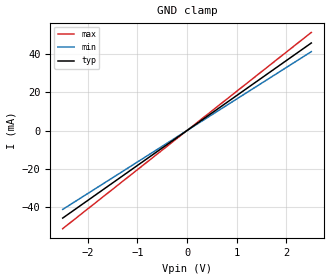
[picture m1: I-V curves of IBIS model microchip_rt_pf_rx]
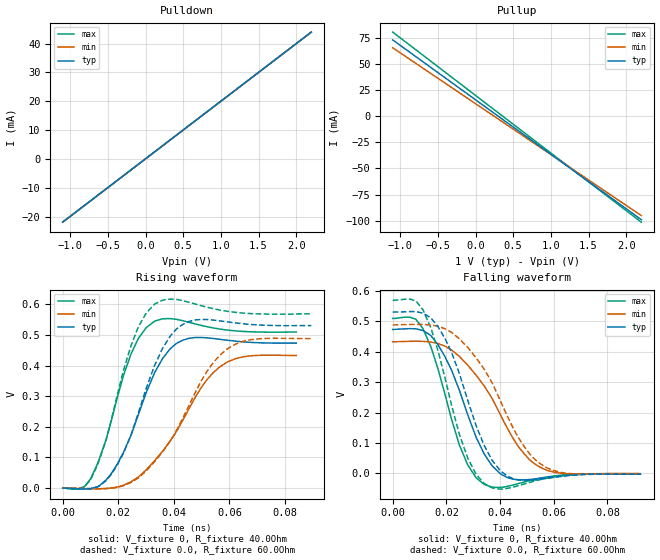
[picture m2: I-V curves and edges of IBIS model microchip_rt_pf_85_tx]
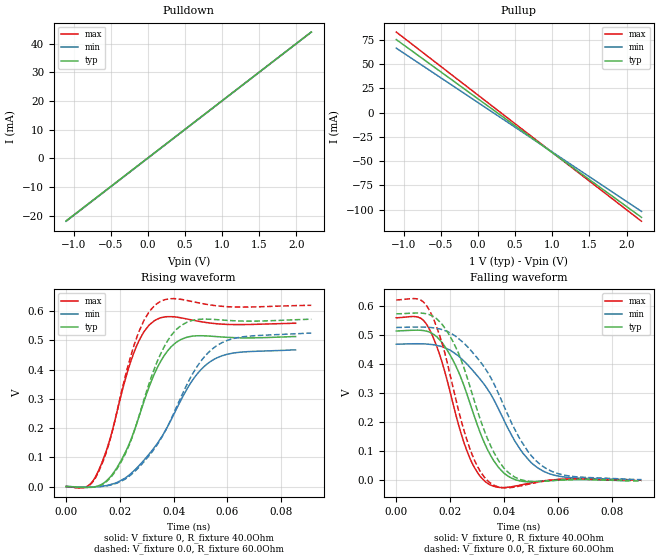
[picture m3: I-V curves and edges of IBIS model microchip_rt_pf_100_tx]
|   Microchip RT PF SerDes IBIS-AMI Model
[IBIS Ver]   6.0
[Disclaimer] THIS IBIS MODEL HAS BEEN CREATED BY THE SIGNAL
   INTEGRITY SOFTWARE SPICE WRAPPING PROCESS.
   THESE IBIS MODELS AREPROVIDED "AS IS" WITH NO
   WARRANTY WHATSOEVER AND SIGNAL INTEGRITY SOFTWARE
   SPECIFICALLY DISCLAIMS ANY IMPLIED WARRANTIES OF
   MERCHANTABILITY, FITNESS FOR A PARTICULAR PURPOSE,
   OR AGAINST INFRINGEMENT.
[File Name]  microchip_rt_pf.ibs
[Date]   Sep/20/2022
[File Rev]   1.0
[Source]   SPISim LLC, Generated by SPIBPro
[Notes]   Revision 1.0 - Sep/20/2022
|   - Passes IBISCHK6 V6.1.4 with 0 Errors and 0 Warnings.
[Copyright]  Copyright 2022, SPISim LLC, All Rights Reserved.
|   COMPONENT: microchip_rt_pf_serdes
[Component] microchip_rt_pf_serdes
[Manufacturer]  microchip
[Package]
R_pkg   0.001m  NA NA
L_pkg   0.000nH NA NA
C_pkg   0.000pF NA NA
[Pin] signal_name   model_name   R_pin L_pin C_pin
1   microchip_rt_pf_rx_p   microchip_rt_pf_rx   NA   NA   NA
2   microchip_rt_pf_rx_n   microchip_rt_pf_rx   NA   NA   NA
3   microchip_rt_pf_85_tx_p   microchip_rt_pf_85_tx   NA   NA   NA
4   microchip_rt_pf_85_tx_n   microchip_rt_pf_85_tx   NA   NA   NA
5   microchip_rt_pf_100_tx_p   microchip_rt_pf_100_tx   NA   NA   NA
6   microchip_rt_pf_100_tx_n   microchip_rt_pf_100_tx   NA   NA   NA
7   microchip_rt_pf_150_tx_p   microchip_rt_pf_150_tx   NA   NA   NA
8   microchip_rt_pf_150_tx_n   microchip_rt_pf_150_tx   NA   NA   NA
9   microchip_rt_pf_180_tx_p   microchip_rt_pf_180_tx   NA   NA   NA
10   microchip_rt_pf_180_tx_n   microchip_rt_pf_180_tx   NA   NA   NA
11   microchip_rt_pf_150_400tx_p   microchip_rt_pf_150_400_tx  NA   NA   NA
12   microchip_rt_pf_150_400tx_n   microchip_rt_pf_150_400_tx  NA   NA   NA
13   microchip_rt_pf_150_800tx_p   microchip_rt_pf_150_800_tx  NA   NA   NA
14   microchip_rt_pf_150_800tx_n   microchip_rt_pf_150_800_tx  NA   NA   NA
15   microchip_rt_pf_180_400tx_p   microchip_rt_pf_180_400_tx  NA   NA   NA
16   microchip_rt_pf_180_400tx_n   microchip_rt_pf_180_400_tx  NA   NA   NA
17   microchip_rt_pf_180_800tx_p   microchip_rt_pf_180_800_tx  NA   NA   NA
18   microchip_rt_pf_180_800tx_n   microchip_rt_pf_180_800_tx  NA   NA   NA
[Diff Pin] inv_pin  vdiff tdelay_typ tdelay_min tdelay_max
1   2   0.0   na   na   na
3   4   0.0   na   na   na
5   6   0.0   na   na   na
7   8   0.0   na   na   na
9   10   0.0   na   na   na
11   12   0.0   na   na   na
13   14   0.0   na   na   na
15   16   0.0   na   na   na
17   18   0.0   na   na   na
| Models and submodels in the file (9): microchip_rt_pf_rx (Input), microchip_rt_pf_85_tx (Output), microchip_rt_pf_100_tx (Output), microchip_rt_pf_150_tx (Output), microchip_rt_pf_180_tx (Output), microchip_rt_pf_150_400_tx (Output), microchip_rt_pf_150_800_tx (Output), microchip_rt_pf_180_400_tx (Output), microchip_rt_pf_180_800_tx (Output)
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|   MODEL: microchip_rt_pf_rx
[Model]   microchip_rt_pf_rx
Model_type Input
Vinl = .05
Vinh = .05
|   typ   min   max
C_comp   0.7pF 0.7pF 0.7pF
[Temperature Range]  65   125  -40
[Voltage Range]   1.0  1.0  1.0
[GND Clamp]
-2.5V     -45.5mA    -41mA      -51mA
0V        0A         0A         0A
2.5V      45.5mA     41mA       51mA
[Algorithmic Model]
Executable Linux_gcc5.4_64   MPF300T-RX_LX64.so   MPF300T-RX.ami
Executable Windows_VisualStudio7.1.3088_64  MPF300T-RX_WIN64.dll  MPF300T-RX.ami
[End Algorithmic Model]
|   MODEL microchip_rt_pf_85_tx
[Model] microchip_rt_pf_85_tx
Model_type   Output
Polarity   Non-Inverting
Enable   Active-High
Vmeas = 0.5
|   typ   min   max
C_comp   0.407p  0.407p  0.407p
[Voltage Range]   1.0  0.9  1.1
[Temperature Range]   60   100   0
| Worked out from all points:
|   slope of the pulldown table from 0 to 0.15 V, typ, clamps not added: 50.1 ohm
|   slope of the pullup table from 0 to 0.15 V, typ, clamps not added: 19.2 ohm
|   rising waveform, V_fixture 0, R_fixture 40.0Ohm: 20-80 % time 12.6ps typ, 18.5ps min, 9.98ps max; typ from 0 V to 0.473 V
|   rising waveform, V_fixture 0.0, R_fixture 60.0Ohm: 20-80 % time 12.9ps typ, 18.6ps min, 10.3ps max; typ from 0 V to 0.531 V
|   falling waveform, V_fixture 0, R_fixture 40.0Ohm: 20-80 % time 12.7ps typ, 18.2ps min, 10ps max; typ from 0.473 V to -0.002 V
|   falling waveform, V_fixture 0.0, R_fixture 60.0Ohm: 20-80 % time 13ps typ, 18.2ps min, 10.4ps max; typ from 0.531 V to -0.003 V
[Pullup]
|   X   TYP   MIN   MAX
-1.1V     72.92mA    65.4mA     80.38mA
1.01V     -37.03mA   -37.25mA   -35.88mA
1.089V    -41.13mA   -41.08mA   -40.2mA
2.2V      -99.03mA   -95.13mA   -101.4mA
[Pulldown]
|   X   TYP   MIN   MAX
-1.1V     -21.92mA   -21.97mA   -21.95mA
1.033V    20.68mA    20.66mA    20.67mA
1.066V    21.35mA    21.34mA    21.34mA
2.2V      44mA       44mA       44mA
[Ramp]
R_load = 50.0Ohm
|   typ   min   max
dV/dt_r   2.84E-1V/1.26E-2ns   2.60E-1V/1.85E-2ns   3.06E-1V/9.91E-3ns
dV/dt_f   2.86E-1V/1.27E-2ns   2.60E-1V/1.81E-2ns   3.07E-1V/9.95E-3ns
[Rising Waveform]
V_fixture   = 0
V_fixture_min = 0
V_fixture_max = 0
R_fixture   = 40.0Ohm
|   Time   V(typ)   V(min)   V(max)
0s        0V         0V         0V
10.09ps   -1.679mV   -2.197mV   30.72mV
17.54ps   47.9mV     325.7uV    221.3mV
24.6ps    172.8mV    20.57mV    438.1mV
33.05ps   376.5mV    88.93mV    545mV
41.5ps    475.3mV    193.6mV    550.1mV
49.84ps   491.8mV    327.8mV    531.3mV
56.35ps   486.1mV    394.6mV    519.6mV
65.4ps    477.3mV    429.3mV    511.4mV
84.09ps   473.4mV    433mV      509.7mV
[Rising Waveform]
V_fixture   = 0.0
V_fixture_min = 0.0
V_fixture_max = 0.0
R_fixture   = 60.0Ohm
|   Time   V(typ)   V(min)   V(max)
0s        0V         0V         0V
10.09ps   -2.194mV   -2.26mV    28.04mV
17.54ps   45.13mV    -379.2uV   223.7mV
24.6ps    173.5mV    18.3mV     465.3mV
33.05ps   399.9mV    85.68mV    600.8mV
38.75ps   497.1mV    154.7mV    617.3mV
43.43ps   535.6mV    231.7mV    611.6mV
51.9ps    550.4mV    380.6mV    590.9mV
59.1ps    543mV      453.8mV    577.6mV
89.49ps   530.8mV    488.3mV    568.9mV
[Falling Waveform]
V_fixture   = 0
V_fixture_min = 0
V_fixture_max = 0
R_fixture   = 40.0Ohm
|   Time   V(typ)   V(min)   V(max)
0s        473.4mV    433mV      509.7mV
8.612ps   475.5mV    434.7mV    507.2mV
11.24ps   470.3mV    434.3mV    477mV
16.85ps   423.5mV    427.1mV    344.6mV
24.81ps   274.2mV    385mV      94.06mV
27.95ps   192.9mV    356mV      27.72mV
34.06ps   64.19mV    288.1mV    -36.36mV
43ps      -14.65mV   143.8mV    -42.29mV
54.85ps   -16.47mV   20.3mV     -16.31mV
92.17ps   -2.492mV   -869.6uV   -1.726mV
[Falling Waveform]
V_fixture   = 0.0
V_fixture_min = 0.0
V_fixture_max = 0.0
R_fixture   = 60.0Ohm
|   Time   V(typ)   V(min)   V(max)
0s        530.8mV    488.3mV    568.9mV
8.612ps   532mV      490.2mV    567.4mV
11.24ps   527.4mV    489.9mV    538.8mV
16.85ps   482.8mV    484mV      404.4mV
24.81ps   328.9mV    442.9mV    129.2mV
27.95ps   240.3mV    414.2mV    50.05mV
34.06ps   92.13mV    343.1mV    -33.29mV
43ps      -10.12mV   182.6mV    -49.1mV
54.85ps   -19.89mV   32.13mV    -21.01mV
92.64ps   -2.906mV   -867.9uV   -1.843mV
[Algorithmic Model]
Executable Linux_gcc5.4_64   MPF300T-TX_LX64.so   MPF300T-TX-R085.ami
Executable Windows_cl18.00.40629_64 MPF300T-TX_WIN64.dll  MPF300T-TX-R085.ami
Executable Windows_cl18.00.40629_32 MPF300T-TX_WIN32.dll  MPF300T-TX-R085.ami
[End Algorithmic Model]
|   MODEL microchip_rt_pf_100_tx
[Model] microchip_rt_pf_100_tx
Model_type   Output
Polarity   Non-Inverting
Enable   Active-High
Vmeas = 0.5
|   typ   min   max
C_comp   0.407p  0.407p  0.407p
[Voltage Range]   1.0  0.9  1.1
[Temperature Range]   60   100   0
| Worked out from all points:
|   slope of the pulldown table from 0 to 0.15 V, typ, clamps not added: 50.1 ohm
|   slope of the pullup table from 0 to 0.15 V, typ, clamps not added: 18 ohm
|   rising waveform, V_fixture 0, R_fixture 40.0Ohm: 20-80 % time 12.9ps typ, 18.6ps min, 10.2ps max; typ from 0 V to 0.513 V
|   rising waveform, V_fixture 0.0, R_fixture 60.0Ohm: 20-80 % time 13.2ps typ, 18.7ps min, 10.6ps max; typ from 0 V to 0.572 V
|   falling waveform, V_fixture 0, R_fixture 40.0Ohm: 20-80 % time 12.9ps typ, 18.2ps min, 10.3ps max; typ from 0.513 V to -0.004 V
|   falling waveform, V_fixture 0.0, R_fixture 60.0Ohm: 20-80 % time 13.3ps typ, 18.3ps min, 10.6ps max; typ from 0.572 V to -0.005 V
[Pullup]
|   X   TYP   MIN   MAX
-1.1V     75.33mA    66.49mA    83.09mA
1.01V     -41.84mA   -41.1mA    -41.62mA
1.089V    -46.2mA    -45.1mA    -46.26mA
2.2V      -107.9mA   -101.8mA   -111.9mA
[Pulldown]
|   X   TYP   MIN   MAX
-1.1V     -21.88mA   -22.01mA   -21.95mA
1.055V    21.14mA    21.1mA     21.12mA
1.089V    21.82mA    21.77mA    21.79mA
2.2V      44mA       44mA       44mA
[Ramp]
R_load = 50.0Ohm
|   typ   min   max
dV/dt_r   3.08E-1V/1.29E-2ns   2.80E-1V/1.86E-2ns   3.35E-1V/1.02E-2ns
dV/dt_f   3.10E-1V/1.29E-2ns   2.80E-1V/1.82E-2ns   3.36E-1V/1.02E-2ns
[Rising Waveform]
V_fixture   = 0
V_fixture_min = 0
V_fixture_max = 0
R_fixture   = 40.0Ohm
|   Time   V(typ)   V(min)   V(max)
0s        0V         0V         0V
10ps      -1.832mV   -1.126mV   19.28mV
17ps      38.74mV    8.035mV    183.8mV
25ps      181.3mV    51.62mV    451.8mV
29ps      290.9mV    90.19mV    529.4mV
33ps      387.8mV    135.4mV    567.6mV
41ps      492.9mV    263.6mV    579.2mV
47ps      514mV      362.8mV    568.9mV
54ps      513.8mV    428.9mV    558.3mV
85.41ps   512.5mV    466.9mV    558mV
[Rising Waveform]
V_fixture   = 0.0
V_fixture_min = 0.0
V_fixture_max = 0.0
R_fixture   = 60.0Ohm
|   Time   V(typ)   V(min)   V(max)
0s        0V         0V         0V
10ps      -2.291mV   -1.468mV   16.69mV
14ps      9.497mV    1.041mV    91.96mV
18ps      47.48mV    8.705mV    218.4mV
26ps      206.7mV    55.67mV    502.3mV
34ps      429.3mV    144mV      626.1mV
43ps      551.4mV    310.4mV    639.4mV
55ps      571.1mV    474.5mV    619mV
65ps      565.7mV    510.7mV    613.4mV
91.26ps   571.7mV    524.5mV    619.4mV
[Falling Waveform]
V_fixture   = 0
V_fixture_min = 0
V_fixture_max = 0
R_fixture   = 40.0Ohm
|   Time   V(typ)   V(min)   V(max)
0s        512.5mV    466.9mV    558mV
8ps       515.3mV    468.5mV    560.4mV
12ps      509.9mV    466.8mV    523.8mV
16ps      483mV      460.7mV    433.7mV
21ps      412.2mV    440mV      264.1mV
27ps      273.3mV    390.8mV    80.8mV
33ps      120.5mV    323.9mV    -6.673mV
41ps      15.29mV    185.2mV    -26.41mV
53ps      -6.188mV   37.82mV    -6.208mV
86.17ps   -3.635mV   321.6uV    -1.579mV
[Falling Waveform]
V_fixture   = 0.0
V_fixture_min = 0.0
V_fixture_max = 0.0
R_fixture   = 60.0Ohm
|   Time   V(typ)   V(min)   V(max)
0s        571.7mV    524.5mV    619.4mV
9ps       574.2mV    526mV      619.4mV
13ps      566.2mV    524.3mV    570.8mV
17ps      535.5mV    517mV      469.8mV
21ps      476.6mV    500.2mV    320.5mV
27ps      331.3mV    452.4mV    115.2mV
35ps      117.3mV    352.6mV    -12.02mV
43ps      14.78mV    191.2mV    -26.61mV
54ps      -5.684mV   48.5mV     -6.444mV
91ps      -4.667mV   501.9uV    -1.775mV
[Algorithmic Model]
Executable Linux_gcc5.4_64   MPF300T-TX_LX64.so   MPF300T-TX-R100.ami
Executable Windows_cl18.00.40629_64 MPF300T-TX_WIN64.dll  MPF300T-TX-R100.ami
Executable Windows_cl18.00.40629_32 MPF300T-TX_WIN32.dll  MPF300T-TX-R100.ami
[End Algorithmic Model]
